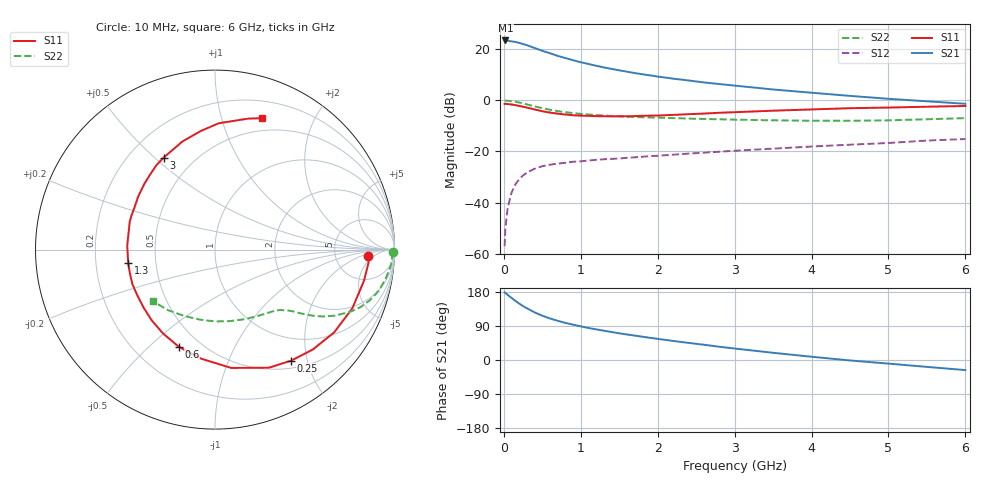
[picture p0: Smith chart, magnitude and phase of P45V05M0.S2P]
! SIEMENS Small Signal Semiconductors
! BFP182
! Si NPN RF Bipolar Junction Transistor in SOT143
! VCE = 5 V  IC = 5 mA
! Common Emitter S-Parameters:  March  1996
# GHz  S  MA  R  50
!  f  S11  S21  S12  S22
! GHz  MAG  ANG  MAG  ANG  MAG  ANG  MAG  ANG
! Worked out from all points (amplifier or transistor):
!   36 points, 10 MHz to 6 GHz, reference 50 ohm
!   highest |S21| = 23.5 dB at 20 MHz (marker M1)
!   |S21| within 3 dB of that: start of sweep to 404 MHz
!   unconditionally stable (mu >= 1): 1.621 GHz to 5.592 GHz
!   at 250 MHz: K = 0.21, MSG = 25.7 dB, |S12| = -29.4 dB
!   at 1.4 GHz: K = 0.91, MSG = 17.6 dB, |S12| = -22.9 dB
!   at 6 GHz: K = 0.94, MSG = 6.9 dB, |S12| = -15.1 dB
!   lowest NFmin = 1.20 dB at 450 MHz
!   S11 on the Smith chart (normalised r, x): 10 MHz: 12, -3; 250 MHz: 0.61, -1.73; 600 MHz: 0.38, -0.62; 1.3 GHz: 0.34, -0.07; 3 GHz: 0.34, +0.54; 6 GHz: 0.37, +1.36
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0.01  0.8528 -2.5  14.78 178.4  0.0014 89.7  0.991 -0.9
0.02  0.8588 -4.7  14.92 177.0  0.0032 86.0  0.9886 -1.9
0.05  0.8481 -11.8  14.74 171.7  0.0078 86.1  0.9844 -4.9
0.15  0.8083 -34.8  13.94 156.1  0.0227 71.3  0.941 -14.1
0.2  0.7791 -45.6  13.39 148.8  0.0287 66.5  0.9087 -18.0
0.25  0.7504 -55.5  12.68 142.2  0.034 61.6  0.8725 -21.5
0.3  0.7236 -65.4  12.06 136.5  0.0385 57.3  0.8336 -24.4
0.4  0.6655 -82.2  10.62 125.6  0.046 51.3  0.7639 -28.8
0.5  0.6127 -97.2  9.34 116.9  0.0515 45.6  0.7057 -31.9
0.6  0.5779 -110.4  8.381 109.6  0.0551 42.4  0.6565 -34.1
0.7  0.5497 -121.8  7.44 103.4  0.0579 39.5  0.6174 -35.7
0.8  0.5291 -131.7  6.754 97.9  0.06 37.7  0.5872 -37.0
1  0.5024 -149.4  5.58 88.7  0.0642 35.5  0.5448 -38.9
1.1  0.4989 -157.3  5.166 84.5  0.0665 34.6  0.5288 -39.9
1.3  0.4893 -171.5  4.428 77.3  0.0704 33.7  0.505 -41.9
1.7  0.493 166.4  3.433 64.5  0.0769 33.3  0.4737 -46.3
2.2  0.5201 145.3  2.667 50.3  0.0865 32.7  0.45 -53.2
3  0.5872 119.1  1.949 30.3  0.1034 30.9  0.4204 -67.5
3.5  0.629 106.8  1.637 19.0  0.1137 28.8  0.4072 -77.9
4.5  0.7037 88.4  1.226 -1.2  0.1359 24.2  0.3993 -102.2
5.5  0.7522 75.9  0.96 -18.2  0.1636 19.1  0.4275 -127.9
6  0.7779 70.3  0.859 -26.6  0.1754 14.8  0.4498 -140.4
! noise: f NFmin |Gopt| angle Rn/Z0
0.45  1.2  0.27  37  0.3
0.9  1.3  0.25  75  0.23
1.8  1.9  0.21  145  0.2
